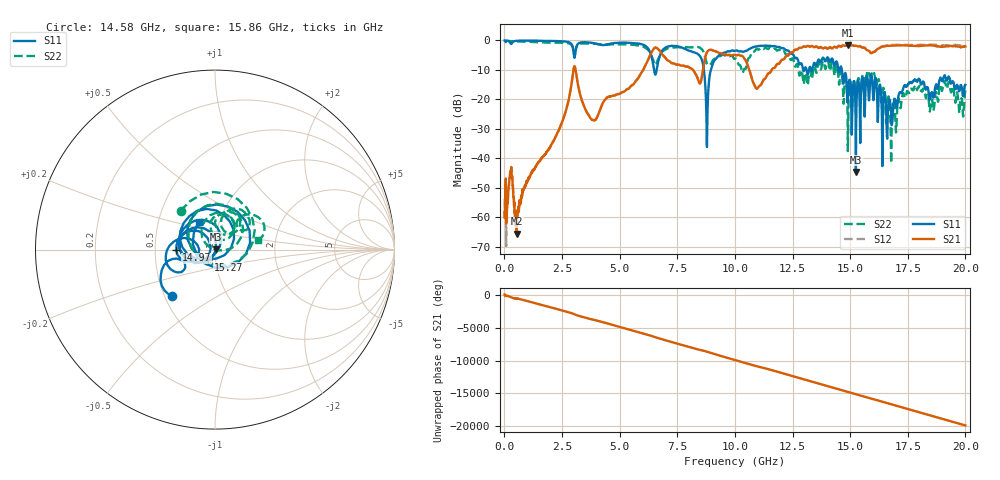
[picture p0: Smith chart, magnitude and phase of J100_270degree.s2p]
!Keysight Technologies,N5222A,MY51421036,A.10.65.16
!Date: Friday, March 31, 2023 14:46:50
!Correction: S11(Full 2 Port(1,2))
!S21(Full 2 Port(1,2))
!S12(Full 2 Port(1,2))
!S22(Full 2 Port(1,2))
!S2P File: Measurements: S11, S21, S12, S22:
# Hz S  dB  R 50
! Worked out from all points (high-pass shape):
!   2000 points, 10 MHz to 20 GHz, reference 50 ohm
!   highest |S21| = -1.60 dB at 14.9 GHz (marker M1); lowest = -65.5 dB at 530 MHz (marker M2)
!   |S21| within 3 dB of the highest: 8.756 GHz to 9.452 GHz (696 MHz wide, 7.64 % of centre); 12.37 GHz to end of sweep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
!   lowest |S11| = -44.6 dB at 15.25 GHz (marker M3), VSWR 1.01, Z = 50.6 + j0.202 ohm
!   |S11| at or under -10 dB: 6.493 GHz to 6.605 GHz (111.7 MHz wide, 1.71 % of centre); 8.655 GHz to 8.959 GHz (303.8 MHz wide, 3.45 % of centre); 14.64 GHz to end of sweep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
!   |S22| runs from -41.6 to -0.1 dB; largest |S21 - S12| = 0.068
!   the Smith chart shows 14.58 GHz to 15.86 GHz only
!   S11 on the Smith chart (normalised r, x): 14.58 GHz: 0.55, -0.32; 14.97 GHz: 0.65, -0.00; 15.27 GHz: 0.92, -0.11; 15.86 GHz: 0.80, +0.26
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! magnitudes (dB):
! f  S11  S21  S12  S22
! 10 MHz  0.0  -58.3  -53.7  -0.1
! 280 MHz  -1.2  -44.2  -43.8  -0.3
! 530 MHz  -0.2  -65.5  -61.3  -0.3
! 3.02 GHz  -5.2  -9.1  -9.1  -3.8
! 3.35 GHz  -0.7  -20.2  -20.1  -1.1
! 3.93 GHz  -1.1  -27.1  -27.0  -1.2
! 6.68 GHz  -6.9  -3.0  -3.0  -6.2
! 8.4 GHz  -4.7  -13.3  -13.2  -2.3
! 8.8 GHz  -29.2  -3.9  -3.8  -8.2
! 9.11 GHz  -6.8  -3.6  -3.6  -6.3
! 10.01 GHz  -3.5  -5.0  -5.0  -6.2
! 10.97 GHz  -2.0  -16.3  -16.3  -2.9
! 13.34 GHz  -10.3  -1.9  -1.8  -13.1
! 14.58 GHz  -9.1  -2.1  -2.0  -10.8
! 14.9 GHz  -20.4  -1.6  -1.5  -37.5
! 14.97 GHz  -13.3  -1.8  -1.7  -14.3
! 15.25 GHz  -44.6  -1.8  -1.7  -19.7
! 15.27 GHz  -23.3  -1.9  -1.7  -20.2
! 15.86 GHz  -14.9  -4.0  -3.8  -12.1
! 16.67 GHz  -21.3  -1.8  -1.6  -19.1
! 17.78 GHz  -13.4  -1.9  -1.5  -16.0
! 20 GHz  -15.1  -2.1  -1.6  -16.9
